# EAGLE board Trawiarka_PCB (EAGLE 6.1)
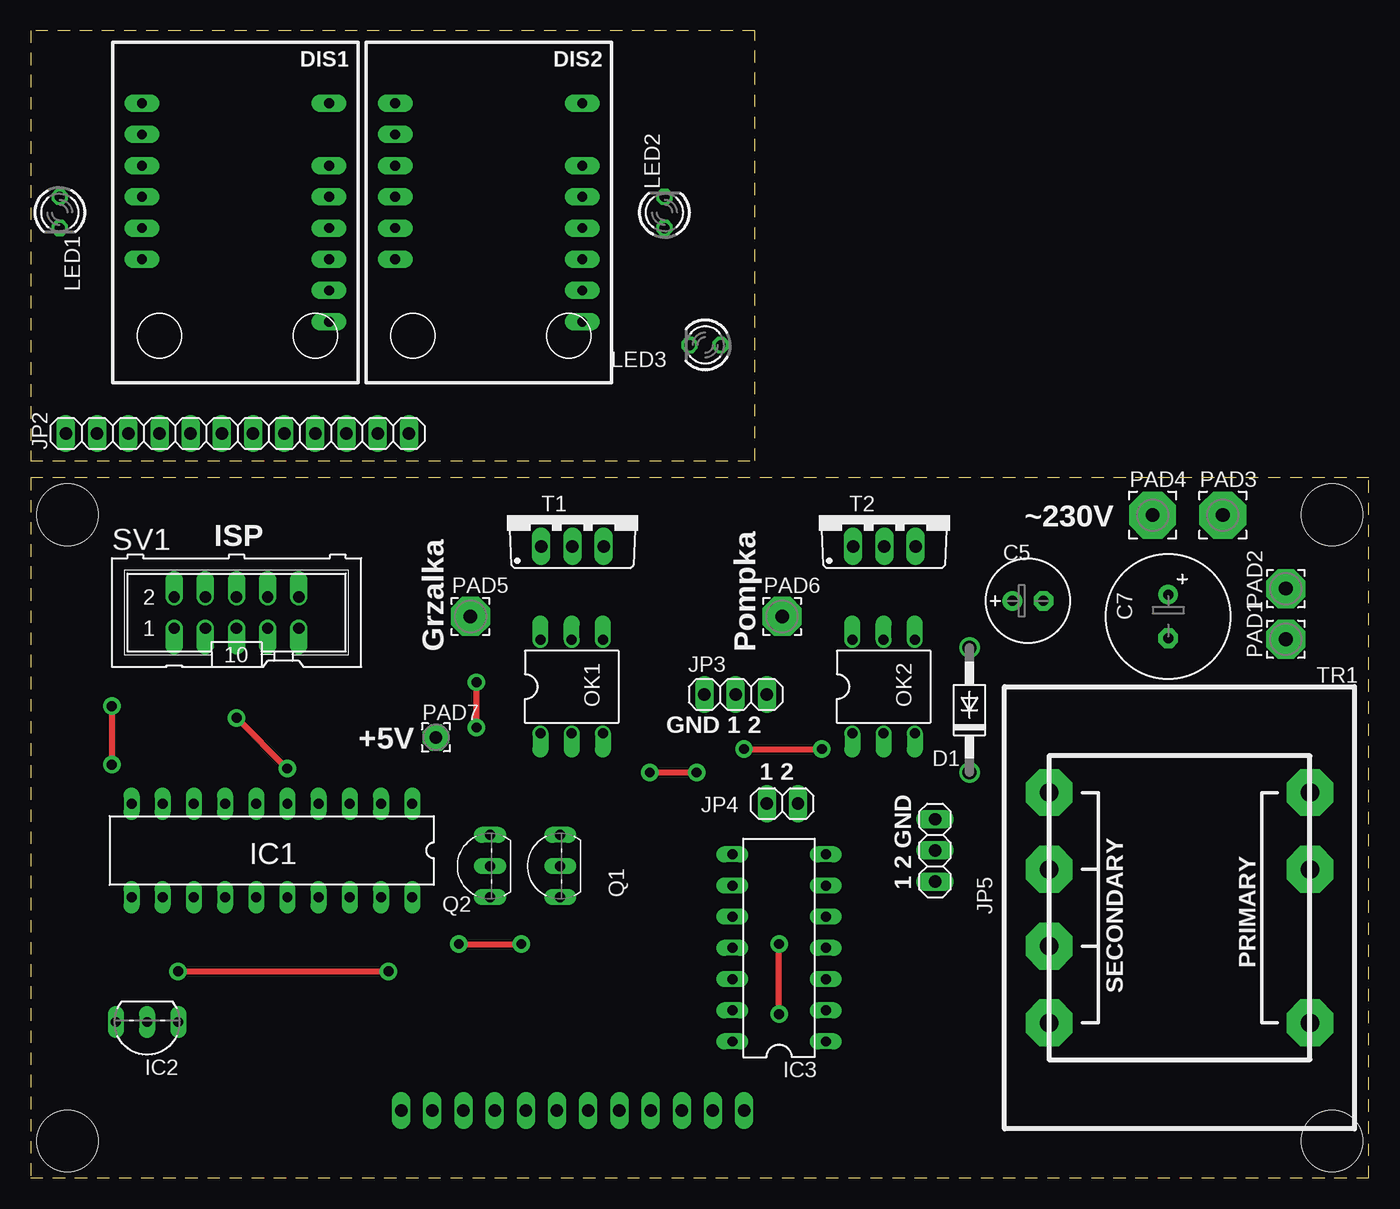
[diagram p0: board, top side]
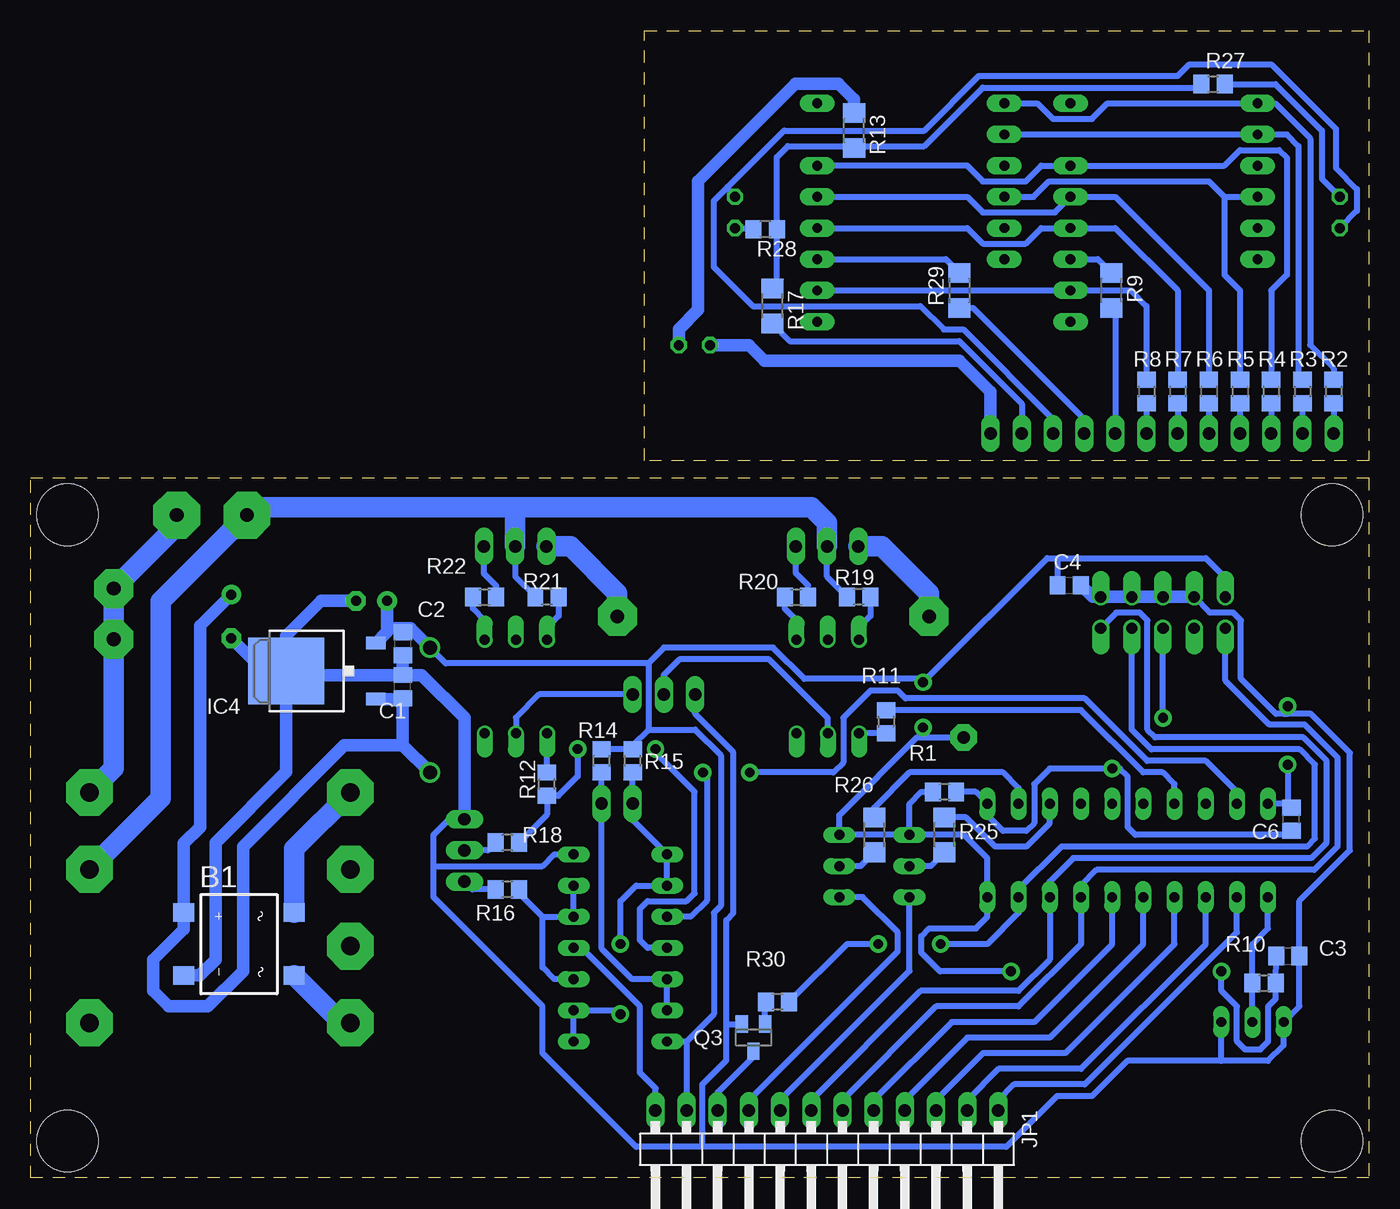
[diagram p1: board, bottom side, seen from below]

Size 109 x 93.42 mm. Coordinates in mm from the lower left corner, seen from the top.
Outline: 0,0 109,0 109,57 0,57 0,0
Outline: 59,58.42 59,93.42 0,93.42 0,58.42 59,58.42
Copper layers (1*16): Top 0.035mm / dielectric 1.5mm / Bottom 0.035mm
Design rules: minimum track width 20mil, minimum drill 24mil, track to track 8mil, track to pad 8mil, pad to pad 8mil, via to via 8mil, smd to smd 8mil, copper to edge 10mil, drill to drill 8mil, minimum pad ring 10mil, minimum via ring 8mil, stop-mask expansion 4mil, vias tented up to drill 0mil, thermal gap 10mil
Holes 5 mm at 3,54 3,3 106,3 106,54

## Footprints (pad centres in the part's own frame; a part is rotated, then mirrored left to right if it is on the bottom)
DFS = smd 1.5 x 1.7: + -2.55,-4.5; - 2.55,-4.5; AC1 -2.55,4.5; AC2 2.55,4.5
C0805 = smd 1.3 x 1.5: 1 -0.95,0; 2 0.95,0
E2,5-7 = drill 0.813 pad 1.6: + -1.27,0 | drill 0.813 pad 1.6 octagon: - 1.27,0
E3,5-10 = drill 0.813 pad 1.6: + -1.778,0 | drill 0.813 pad 1.6 octagon: - 1.778,0
DO41-10 = drill 1.118: A 5.08,0; C -5.08,0
SA08-11XX = drill 0.8 pad 1.422 long: 1 2.38,22.74; 2 2.38,20.2; 3 2.38,17.66; 4 2.38,15.12; 5 2.38,12.58; 6 2.38,10.04; 9 17.62,4.96; 10 17.62,7.5; 11 17.62,10.04; 12 17.62,12.58; 13 17.62,15.12; 14 17.62,17.66; 16 17.62,22.74
DIL20 = drill 0.813 long: 1 -11.43,-3.81; 2 -8.89,-3.81; 3 -6.35,-3.81; 4 -3.81,-3.81; 5 -1.27,-3.81; 6 1.27,-3.81; 7 3.81,-3.81; 8 6.35,-3.81; 9 8.89,-3.81; 10 11.43,-3.81; 11 11.43,3.81; 12 8.89,3.81; 13 6.35,3.81; 14 3.81,3.81; 15 1.27,3.81; 16 -1.27,3.81; 17 -3.81,3.81; 18 -6.35,3.81; 19 -8.89,3.81; 20 -11.43,3.81
TO92- = drill 0.813 long: 1 -2.54,0; 2 0,0; 3 2.54,0
DIL14 = drill 0.813 long: 1 -7.62,-3.81; 2 -5.08,-3.81; 3 -2.54,-3.81; 4 0,-3.81; 5 2.54,-3.81; 6 5.08,-3.81; 7 7.62,-3.81; 8 7.62,3.81; 9 5.08,3.81; 10 2.54,3.81; 11 0,3.81; 12 -2.54,3.81; 13 -5.08,3.81; 14 -7.62,3.81
TO252 = smd 1 x 1.6: 1 -2.28,-4.8; 2 2.28,-4.8 | smd 5.4 x 6.2: 3 0,2.5
1X12/90 = drill 1.016 long: 1 -13.97,-3.81; 2 -11.43,-3.81; 3 -8.89,-3.81; 4 -6.35,-3.81; 5 -3.81,-3.81; 6 -1.27,-3.81; 7 1.27,-3.81; 8 3.81,-3.81; 9 6.35,-3.81; 10 8.89,-3.81; 11 11.43,-3.81; 12 13.97,-3.81
1X12 = drill 1.016 long: 1 -13.97,0; 2 -11.43,0; 3 -8.89,0; 4 -6.35,0; 5 -3.81,0; 6 -1.27,0; 7 1.27,0; 8 3.81,0; 9 6.35,0; 10 8.89,0; 11 11.43,0; 12 13.97,0
1X03 = drill 1.016 long: 1 -2.54,0; 2 0,0; 3 2.54,0
1X02 = drill 1.016 long: 1 -1.27,0; 2 1.27,0
LED3MM = drill 0.813 octagon: A -1.27,0; K 1.27,0
DIL06 = drill 0.813 offset: 1 -2.54,-3.81; 2 0,-3.81; 3 2.54,-3.81; 4 2.54,3.81; 5 0,3.81; 6 -2.54,3.81
3,17/1,1 = drill 1.118 pad 3.175 octagon: 1 0,0
3,81/1,1 = drill 1.118 pad 3.81 octagon: 1 0,0
2,15/1,0 = drill 1.016 pad 2.159 octagon: 1 0,0
TO92-EBC = drill 0.813 long: B 0,-1.27; C -2.54,-1.27; E 2.54,-1.27
SOT23 = smd 1 x 1.4: 1 -0.95,-1.1; 2 0.95,-1.1; 3 0,1.1
R0805 = smd 1.3 x 1.5: 1 -0.95,0; 2 0.95,0
R1206 = smd 1.6 x 1.803: 1 -1.422,0; 2 1.422,0
ML10 = drill 0.914 offset: 1 -5.08,-1.27; 2 -5.08,1.27; 3 -2.54,-1.27; 4 -2.54,1.27; 5 0,-1.27; 6 0,1.27; 7 2.54,-1.27; 8 2.54,1.27; 9 5.08,-1.27; 10 5.08,1.27
TO220BV = drill 1.016 long: G 2.54,-2.54; T1 -2.54,-2.54; T2 0,-2.54
EI36 = drill 1.5 pad 3.81 octagon: NC 27.375,24.875; PR1 8.625,24.875; PR2 14.875,24.875; SEC1 8.625,3.625; SEC2 14.875,3.625; SEC3 21.125,3.625; SEC4 27.375,3.625

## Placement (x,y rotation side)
B1  DF06S  [DFS]  92.03,19.05 270 bottom
C1  100n  [C0805]  78.69,40.01 90 bottom
C2  100n  [C0805]  78.69,43.5 270 bottom
C3  100n  [C0805]  6.61,18.08 0 bottom
C4  100n  [C0805]  24.4,48.26 0 bottom
C5  470u  [E2,5-7]  81.23,46.99 0 top
C6  100n  [C0805]  6.3,29.21 90 bottom
C7  1000u  [E3,5-10]  92.66,45.72 270 top
D1  1N4007  [DO41-10]  76.47,38.1 90 top
DIS1  [SA08-11XX]  6.68,64.77 0 top
DIS2  [SA08-11XX]  27.32,64.77 0 top
IC1  ATtiny2313  [DIL20]  19.64,26.67 180 top
IC2  DS18B20  [TO92-]  9.48,12.7 180 top
IC3  4093N  [DIL14]  60.96,18.73 90 top
IC4  78M05  [TO252]  85.68,41.27 90 bottom
JP1  [1X12/90]  44.15,1.7 180 bottom
JP2  [1X12]  16.84,60.62 0 top
JP3  LED  [1X03]  57.42,39.37 0 top
JP4  BTN  [1X02]  61.23,30.48 180 top
JP5  LED-BTN  [1X03]  73.66,26.67 90 top
LED1  [LED3MM]  2.37,78.62 270 top
LED2  [LED3MM]  51.63,78.62 90 top
LED3  [LED3MM]  54.94,67.83 180 top
OK1  MOC3041  [DIL06]  44.07,40.01 0 top
OK2  MOC3041  [DIL06]  69.47,40.01 0 top
PAD1  [3,17/1,1]  102.23,43.87 90 top
PAD2  [3,17/1,1]  102.23,47.99 90 top
PAD3  [3,81/1,1]  97.11,53.98 0 top
PAD4  [3,81/1,1]  91.39,53.98 0 top
PAD5  [3,17/1,1]  35.81,45.72 0 top
PAD6  [3,17/1,1]  61.22,45.72 0 top
PAD7  VCC  [2,15/1,0]  33.02,35.88 0 top
Q1  BC558C  [TO92-EBC]  41.87,25.4 90 top
Q2  BC558C  [TO92-EBC]  36.15,25.4 90 top
Q3  BC846  [SOT23]  50.12,11.43 180 bottom
R1  10k  [R0805]  34.56,31.43 180 bottom
R2  330  [R0805]  2.87,64.04 270 bottom
R3  330  [R0805]  5.41,64.04 270 bottom
R4  330  [R0805]  7.95,64.04 270 bottom
R5  330  [R0805]  10.49,64.04 270 bottom
R6  330  [R0805]  13.03,64.04 270 bottom
R7  330  [R0805]  15.57,64.04 270 bottom
R8  330  [R0805]  18.11,64.04 270 bottom
R9  0  [R1206]  20.97,72.27 270 bottom
R10  4k7  [R0805]  8.53,15.88 0 bottom
R11  220  [R0805]  39.32,37.15 270 bottom
R12  220  [R0805]  66.94,32.07 90 bottom
R13  470  [R1206]  41.92,85.29 270 bottom
R14  4k7  [R0805]  62.5,33.97 90 bottom
R15  4k7  [R0805]  59.96,33.97 90 bottom
R16  470  [R0805]  70.17,23.5 180 bottom
R17  0  [R1206]  48.59,71 270 bottom
R18  470  [R0805]  70.17,27.3 180 bottom
R19  220  [R0805]  41.55,47.32 180 bottom
R20  220  [R0805]  46.62,47.29 0 bottom
R21  220  [R0805]  66.94,47.32 180 bottom
R22  220  [R0805]  72.03,47.29 0 bottom
R25  4k7  [R1206]  34.56,27.94 270 bottom
R26  4k7  [R1206]  40.28,27.94 270 bottom
R27  470  [R0805]  12.69,89.08 0 bottom
R28  470  [R0805]  49.16,77.25 180 bottom
R29  0  [R1206]  33.35,72.27 90 bottom
R30  4k7  [R0805]  48.16,14.34 180 bottom
SV1  ISP  [ML10]  16.77,46.04 0 top
T1  BT136  [TO220BV]  44.13,53.98 0 top
T2  BT136  [TO220BV]  69.53,53.98 0 top
TR1  [EI36]  79.33,40.01 270 top

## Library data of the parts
B1 = rectifier
C1-C7 R1-R22 R25-R30 = rcl
D1 = diode
DIS1 DIS2 = led-7-segment
IC1 = atmel
IC2 = maxim
IC3 = 40xx
IC4 = linear
JP1-JP5 = pinhead
LED1-LED3 = led
OK1 OK2 = optocoupler
PAD1-PAD7 = wirepad
Q1 Q2 = transistor-pnp
Q3 = transistor-npn
SV1 = con-harting-ml-2
T1 T2 = triac
TR1 = trafo

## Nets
A: DIS1.1 DIS2.1 R2.1
B: DIS1.14 DIS2.14 R4.1
C: DIS1.12 DIS2.12 R7.1
D: DIS1.10 DIS2.10 R8.1
E: DIS1.4 DIS2.4 R5.1
F: DIS1.2 DIS2.2 R3.1
G: DIS1.13 DIS2.13 R6.1
GND: B1.- C1.2 C2.2 C3.2 C4.2 C5.- C6.2 C7.- IC1.10 IC2.1 IC2.3 IC3.7 IC4.3 JP3.1 JP5.3 Q3.2 SV1.4 SV1.6 SV1.8 SV1.10
N$1: IC1.11 IC2.2 R10.1
N$2: OK1.6 R19.1
N$3: R20.2 T1.G
N$4: B1.+ C1.1 C7.+ D1.C IC4.1
N$5: JP3.2 OK1.2
N$6: B1.AC1 TR1.SEC1
N$7: B1.AC2 TR1.SEC4
N$8: C6.1 IC1.1 R1.1 SV1.5
N$9: JP3.3 OK2.2
N$10: OK1.1 R11.2
N$11: LED3.A R13.1
N$12: OK2.1 R12.2
N$13: IC3.11 R12.1 R18.1
N$14: JP2.8 R9.2
N$15: IC3.3 IC3.5 IC3.6 R16.1
N$16: JP5.2 R18.2
N$17: JP2.1 R2.2
N$18: OK1.4 R20.1
N$19: R22.2 T2.G
N$20: IC3.1 IC3.2 IC3.8 IC3.9 JP4.2 R15.1
N$21: OK2.6 R21.1
N$22: OK2.4 R22.1
N$23: PAD6.1 T2.T1
N$24: PAD5.1 T1.T1
N$25: IC3.12 IC3.13 JP4.1 R14.1
N$26: JP2.9 R29.1
N$27: JP5.1 R16.2
N$28: JP2.12 LED3.K
N$29: IC3.4 JP1.12
N$30: Q2.B R25.2
N$31: Q1.B R26.2
N$32: Q3.1 R30.2
N$33: JP2.11 R17.2
N$34: IC1.9 IC3.10
N$37: IC1.17 JP1.6 SV1.1
N$38: IC1.18 JP1.7 SV1.9
N$39: PAD4.1 R19.2 R21.2 T1.T2 T2.T2 TR1.PR2
N$40: IC1.7 R11.1
N$41: PAD1.1 PAD2.1 PAD3.1 TR1.PR1
N$42: LED1.A R27.2
N$44: JP2.2 R3.2
N$45: JP2.3 R4.2
N$46: JP2.4 R5.2
N$47: JP2.5 R6.2
N$48: JP2.6 R7.2
N$49: JP2.7 R8.2
N$51: JP2.10 LED1.K LED2.K
N$53: IC1.12 JP1.1
N$54: IC1.13 JP1.2
N$55: IC1.14 JP1.3
N$56: IC1.15 JP1.4
N$57: IC1.16 JP1.5
N$58: JP1.8 Q2.C
N$59: JP1.9 Q1.C
N$65: IC1.3 R25.1
N$66: IC1.2 R26.1
N$68: LED2.A R28.2
N$72: DIS2.11 R29.2
N$73: DIS1.11 R9.1
N$74: R13.2 R17.1 R27.1 R28.1
N$80: JP1.10 Q3.3
N$82: IC1.19 R30.1 SV1.7
VCC: C2.1 C3.1 C4.1 C5.+ D1.A IC1.20 IC3.14 IC4.2 JP1.11 PAD7.1 Q1.E Q2.E R1.2 R10.2 R14.2 R15.2 SV1.2

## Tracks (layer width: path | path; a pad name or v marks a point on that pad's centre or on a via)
A
  Bottom 0.508: DIS2.1 27,87.51 25.73,86.24 22.55,86.24 21.29,87.51 DIS1.1 7.63,87.51 4.78,84.65 4.78,67.83 2.87,65.92 R2.1
B
  Bottom 0.508: DIS2.14 32.72,82.43 31.45,81.16 27.95,81.16 26.68,82.43 DIS1.14 11.76,82.43 10.49,83.7 7.32,83.7 6.68,83.06 6.68,73.54 7.95,72.27 R4.1
C
  Bottom 0.508: DIS2.12 32.72,77.35 31.45,76.08 27.95,76.08 26.68,77.35 DIS1.12 20.65,77.35 15.57,72.27 R7.1
D
  Bottom 0.508: DIS2.10 DIS1.10 19.38,72.27 18.11,71 R8.1
E
  Bottom 0.508: 11.76,79.89 DIS1.4 | DIS2.4 27.32,79.89 26.05,81.16 13.03,81.16 11.76,79.89 | R5.1 10.49,72.27 11.76,73.54 11.76,79.89
F
  Bottom 0.508: DIS2.2 DIS1.2 6.68,84.97 5.73,84.02 5.73,65.31 R3.1
G
  Bottom 0.508: DIS2.13 32.72,79.89 31.45,78.62 25.57,78.62 DIS1.13 20.65,79.89 13.03,72.27 R6.1
GND  (via drill 0.8 pad 1.42)
  Top 0.508: v6.61,38.42 v6.61,33.66
  Bottom 0.508: 12,9.53 8.21,9.53 6.94,10.79 IC2.3 5.66,13.98 C3.2 5.65,17.77 5.65,22.56 1.54,26.67 1.54,34.61 4.71,37.78 6.94,37.78 | IC2.1 12.02,9.54 12,9.53 | SV1.4 12.96,46.04 11.05,46.04 10.41,45.4 10.41,40.64 7.56,37.78 6.94,37.78 | JP3.1 54.88,37.78 51.75,34.66 51.75,21.59 52.34,21 52.34,12.38 | IC1.10 6.62,30.48 6.61,30.46 | v6.61,33.66 6.61,30.46 | 6.61,30.46 C6.2 | v6.61,38.42 6.61,37.8 6.94,37.78 | 54.29,2.54 54.29,7.62 52.34,9.57 52.34,12.38 | 12,9.53 19.68,9.53 22.54,6.67 25.4,6.67 29.53,2.54 54.29,2.54 | Q3.2 52.19,12.53 52.34,12.38 | 54.29,2.54 59.69,2.54 67.31,10.16 67.31,13.97 76.2,22.86 76.2,25.4 | 76.2,25.4 76.2,27.94 74.93,29.21 JP5.3 | IC3.7 66.36,26.35 67.31,25.4 76.2,25.4
  Bottom 1.016: SV1.4 SV1.6 SV1.8 SV1.10 22.5,47.31 C4.2 | B1.- 95.22,16.5 93.94,17.78 93.94,27.3 88.18,33.06 IC4.3 | 88.9,41.27 IC4.3 | 88.9,41.27 89.99,41.27 C7.- | C5.- 85.36,46.99 88.18,44.17 IC4.3 | JP5.3 73.66,37.47 77.15,40.95 C1.2 | C1.2 88.58,40.95 88.9,41.27 | C1.2 C2.2
N$1
  Bottom 0.508: IC1.11 8.21,20.32 9.48,19.05 9.48,15.24 | IC2.2 9.48,15.24 | R10.1 9.48,15.24
N$2
  Bottom 0.508: R19.1 40.59,45.77 41.53,44.83 OK1.6
N$3
  Bottom 0.508: R20.2 45.67,48.26 46.67,49.26 T1.G
N$4
  Bottom 1.016: IC4.1 78.75,38.99 C1.1 78.69,35.24 | C7.+ 95.2,44.96 95.2,28.58 96.53,27.25 B1.+ 96.53,20.27 99.02,17.78 99.02,15.24 97.75,13.97 94.57,13.97 91.71,16.83 91.71,26.99 83.46,35.24 78.69,35.24 | 78.69,35.24 D1.C
N$5
  Bottom 0.508: OK1.2 44.07,37.45 48.85,42.23 56.15,42.23 57.42,40.96 JP3.2
N$6
  Bottom 1.676: B1.AC1 87.53,26.8 TR1.SEC1
N$7
  Bottom 1.676: TR1.SEC4 83.66,12.63 B1.AC2
N$8  (via drill 0.8 pad 1.42)
  Top 0.508: v20.89,33.34 v16.77,37.47
  Bottom 0.508: R1.1 32.02,31.43 IC1.1 31.07,29.53 29.8,28.26 27.89,28.26 27.26,28.89 27.26,32.07 25.99,33.34 v20.89,33.34 20.27,33.34 19.64,32.7 19.64,28.57 19,27.94 6.62,27.94 C6.1 | v16.77,37.47 SV1.5
N$9
  Bottom 0.508: JP3.3 67.58,39.37 69.47,37.48 OK2.2
N$10
  Bottom 0.508: OK1.1 R11.2
N$11
  Bottom 1.016: R13.1 41.92,87.83 43.19,89.1 46.69,89.1 54.62,81.16 54.62,70.68 56.21,69.09 LED3.A
N$12
  Bottom 0.508: OK2.1 66.93,33.03 R12.2
N$13  (via drill 0.8 pad 1.42)
  Top 0.508: v58.1,34.92 v64.45,34.92
  Bottom 0.508: IC3.11 58.74,18.73 59.37,19.37 59.37,21.91 58.74,22.54 55.56,22.54 54.93,23.18 54.93,31.43 58.1,34.61 v58.1,34.92 | v64.45,34.92 64.45,32.7 66.04,31.12 R12.1 66.94,29.58 R18.1
N$14
  Bottom 0.508: JP2.8 20.65,70.53 R9.2
N$15
  Bottom 0.508: IC3.3 66.36,16.19 67.31,17.14 67.31,21.27 | IC3.6 IC3.5 67.31,21.27 | R16.1 69.22,23.18 67.31,21.27
N$16
  Bottom 0.508: JP5.2 71.75,26.67 R18.2
N$17
  Bottom 0.508: R2.2 JP2.1
N$18
  Bottom 0.508: R20.1 47.58,46.35 46.62,45.4 46.62,43.83 OK1.4
N$19
  Bottom 0.508: R22.2 71.08,48.22 72.07,49.21 T2.G
N$20  (via drill 0.8 pad 1.42)
  Top 0.508: v60.96,13.34 v60.96,19.05
  Bottom 0.508: R15.1 JP4.2 59.96,29.16 IC3.8 IC3.9 59.69,23.81 60.96,22.54 v60.96,19.05 | IC3.1 IC3.2 61.28,13.65 v60.96,13.34
N$21
  Bottom 0.508: R21.1 66,45.77 66.93,44.83 OK2.6
N$22
  Bottom 0.508: R22.1 72.97,46.35 72.01,45.39 OK2.4
N$23
  Bottom 1.676: PAD6.1 61.23,45.73 61.23,47.62 65.04,51.44 T2.T1
N$24
  Bottom 1.676: PAD5.1 35.83,45.73 35.83,47.62 39.64,51.44 T1.T1
N$25
  Bottom 0.508: R14.1 JP4.1 62.5,18.68 60.01,16.19 IC3.12 IC3.13
N$26
  Bottom 0.508: JP2.9 23.19,61.79 32.24,70.85 R29.1
N$27
  Bottom 0.508: R16.2 73.03,23.5 JP5.1
N$28
  Bottom 1.016: LED3.K 50.49,67.83 49.23,66.56 33.35,66.56 30.81,64.02 JP2.12
N$29
  Bottom 0.508: IC3.4 64.14,18.73 59.37,13.97 59.37,8.57 58.1,7.3 58.1,5.52 JP1.12
N$30
  Bottom 0.508: Q2.B 35.68,25.4 R25.2
N$31
  Bottom 0.508: Q1.B 41.4,25.4 R26.2
N$32
  Bottom 0.508: Q3.1 49.17,14.28 R30.2
N$33
  Bottom 0.508: JP2.11 28.27,63.06 33.35,68.14 47.15,68.14 R17.2
N$34  (via drill 0.8 pad 1.42)
  Top 0.508: v50.44,33.02 v54.24,33.02
  Bottom 0.508: IC1.9 10.75,31.43 13.29,33.97 18.05,33.97 23.13,39.05 37.73,39.05 38.37,39.69 40.59,39.69 42.81,37.47 42.81,33.82 43.62,33.02 v50.44,33.02 | v54.24,33.02 53.93,32.7 53.93,22.59 55.24,21.27 IC3.10
N$37
  Bottom 0.508: SV1.1 11.69,40.49 8.1,36.91 5.22,36.91 2.54,34.22 2.54,27 4.46,25.08 22.18,25.08 23.45,23.81 IC1.17 23.45,19.05 28.53,13.97 35.24,13.97 42.88,6.34 JP1.6
N$38
  Bottom 0.508: SV1.9 20.57,46.04 18.67,46.04 18.04,45.4 18.04,36.51 17.4,35.88 5.33,35.88 3.43,33.97 3.43,27.3 4.7,26.04 24.09,26.04 25.99,24.13 IC1.18 25.99,17.78 28.53,15.24 36.51,15.24 45.41,6.34 JP1.7
N$39
  Bottom 0.508: T2.T2 69.53,48.96 R21.2 | T1.T2 44.13,48.96 R19.2
  Bottom 1.676: 69.48,54.61 69.47,54.59 | 69.48,54.61 90.76,54.61 PAD4.1 98.42,46.95 98.42,30.91 TR1.PR2 | T2.T2 69.53,54.56 69.48,54.61 | 69.48,54.61 45.4,54.61 44.13,53.34 T1.T2
N$40
  Bottom 0.508: IC1.7 15.83,32.07 16.78,33.02 18.37,33.02 23.45,38.1 R11.1
N$41
  Bottom 1.676: PAD3.1 97.11,53.12 PAD2.1 PAD1.1 102.23,33.35 TR1.PR1
N$42
  Bottom 0.508: R27.2 7.61,89.08 3.82,85.29 3.82,81.35 LED1.A
N$44
  Bottom 0.508: R3.2 JP2.2
N$45
  Bottom 0.508: R4.2 JP2.3
N$46
  Bottom 0.508: R5.2 JP2.4
N$47
  Bottom 0.508: R6.2 JP2.5
N$48
  Bottom 0.508: R7.2 JP2.6
N$49
  Bottom 0.508: R8.2 JP2.7
N$51
  Bottom 0.508: JP2.10 25.73,61.79 33.03,69.09 34.62,69.09 36.52,71 50.18,71 53.35,74.17 53.35,79.57 52.24,80.68 | LED1.K 0.96,78.75 0.96,80.53 2.68,82.24 2.68,85.42 7.95,90.69 14.62,90.69 15.57,89.73 31.76,89.73 36.21,85.29 47.64,85.29 52.24,80.68 | LED2.K 52.24,80.5 52.24,80.68
N$53
  Bottom 0.508: IC1.12 10.75,20 23.13,7.62 28.89,7.62 30.18,6.34 JP1.1
N$54
  Bottom 0.508: IC1.13 13.29,19.05 23.45,8.89 30.16,8.89 32.72,6.34 JP1.2
N$55
  Bottom 0.508: IC1.14 15.83,19.05 24.72,10.16 31.43,10.16 35.26,6.34 JP1.3
N$56
  Bottom 0.508: IC1.15 18.37,19.05 25.99,11.43 32.7,11.43 37.8,6.34 JP1.4
N$57
  Bottom 0.508: IC1.16 20.91,19.05 27.26,12.7 33.97,12.7 40.34,6.34 JP1.5
N$58
  Bottom 0.508: Q2.C 37.42,16.87 47.95,6.34 JP1.8
N$59
  Bottom 0.508: Q1.C 41.23,22.86 38.37,20 38.37,18.46 50.49,6.34 JP1.9
N$65
  Bottom 0.508: IC1.3 25.99,28.89 27.89,26.99 30.43,26.99 32.81,29.36 R25.1
N$66
  Bottom 0.508: R26.1 40.28,30.16 37.42,33.02 29.8,33.02 28.53,31.75 IC1.2
N$68
  Bottom 0.508: R28.2 50.22,77.35 LED2.A
N$72
  Bottom 0.508: DIS2.11 34.47,74.81 R29.2
N$73
  Bottom 0.508: DIS1.11 22.09,74.81 R9.1
N$74
  Bottom 0.508: R27.1 13.94,88.78 31.45,88.78 36.21,84.02 41.92,84.02 | R17.1 48.22,72.8 R28.1 48.22,83.12 47.32,84.02 41.92,84.02 | 41.92,84.02 R13.2
N$80
  Bottom 0.508: JP1.10 53.02,5.52 53.02,6.99 50.12,9.89 Q3.3
N$82  (via drill 0.8 pad 1.42)
  Top 0.508: v34.88,19.05 v39.96,19.05
  Bottom 0.508: v34.88,19.05 31.07,19.05 28.53,21.59 IC1.19 28.53,23.5 25.04,26.99 5.02,26.99 4.38,27.62 4.38,33.66 5.63,34.91 17.7,34.91 19.3,36.51 SV1.7 | v39.96,19.05 42.5,19.05 R30.1
VCC  (via drill 0.8 pad 1.42)
  Top 0.508: v12,16.83 v29.15,16.83 | v36.32,36.68 v36.32,40.37
  Bottom 0.508: Q2.E Q1.E 43.13,29.55 36.8,35.88 36.2,35.88 | Q2.E 32.98,27.94 31.07,26.04 IC1.20 31.07,21.25 32.01,20.32 35.81,20.32 36.45,19.68 36.45,18.35 34.92,16.83 v29.15,16.83 | R1.2 36.47,31.43 37.42,30.48 Q2.E | v12,16.83 12,15.24 10.73,13.97 10.73,11.11 10.1,10.48 8.83,10.48 8.19,11.11 8.19,13.97 7.58,14.59 R10.2 C3.1 | SV1.2 11.69,48.88 13.29,50.48 25.35,50.48 | 25.35,50.48 26.2,50.48 36.04,40.64 | C4.1 25.35,50.16 25.35,50.48 | v36.32,40.37 36.04,40.64 | D1.A 75.2,41.91 58.69,41.91 | 58.69,41.91 57.42,43.18 48.53,43.18 45.99,40.64 36.04,40.64 | R15.2 | 58.69,41.91 58.69,36.51 | R15.2 R14.2 | R15.2 59.96,35.24 58.69,36.51 | 58.69,36.51 54.88,36.51 52.77,34.4 52.77,22.16 53.34,21.59 53.34,13.34 55.58,11.1 | 36.2,35.88 PAD7.1 | v36.32,36.68 36.32,36 36.2,35.88 | 55.58,11.1 JP1.11 | 55.58,11.1 57.14,11.1 IC3.14
  Bottom 1.016: C2.1 79.01,44.77 | 79.97,44.77 79.97,44.47 IC4.2 | 79.97,44.77 C5.+ | 79.01,44.77 79.97,44.77 | 79.01,44.77 78.06,44.77 D1.A

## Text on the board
tPlace: ~230V | ISP | Grzalka | Pompka | GND 1 2 | +5V | 1 2 | 1 2 GND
